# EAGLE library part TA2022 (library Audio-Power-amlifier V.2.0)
STEREO 90W (4.) CLASS-TM DIGITAL AUDIO AMPLIFIER DRIVER USING DIGITAL POWER PROCESSING (DPP TM) TECHNOLOGY Source: http://www.tripath.com/audio.htm .. TA2022.pdf
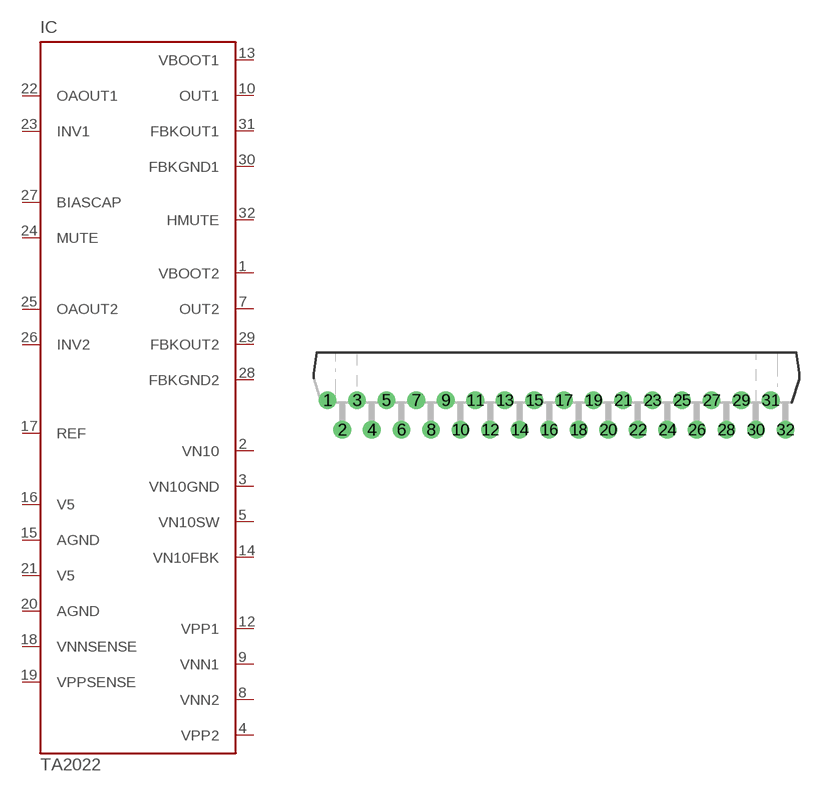
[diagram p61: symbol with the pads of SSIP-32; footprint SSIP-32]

Designator prefix IC

## TA2022 (OC_FARNELL: unknown; OC_NEWARK: unknown)  [SSIP-32]
1  VBOOT2  in
2  VN10  in
3  VN10GND  pwr
4  VPP2  pwr
5  VN10SW  out
7  OUT2  out
8  VNN2  pwr
9  VNN1  pwr
10  OUT1  out
12  VPP1  pwr
13  VBOOT1  in
14  VN10FBK  out
15  AGND  pwr
16  V5  pwr
17  REF  pas
18  VNNSENSE  in
19  VPPSENSE  in
20  AGND  pwr
21  V5  pwr
22  OAOUT1  out
23  INV1  in
24  MUTE  in
25  OAOUT2  out
26  INV2  in
27  BIASCAP  pas
28  FBKGND2  out
29  FBKOUT2  out
30  FBKGND1
31  FBKOUT1  out
32  HMUTE  out

## Footprint SSIP-32 (pad centres in mm)
32-pin SSIP Source: http://www.tripath.com/audio.htm
drill 0.813 pad 1.524: 1 -19.685,2.54; 2 -18.415,0; 3 -17.145,2.54; 4 -15.875,0; 5 -14.605,2.54; 6 -13.335,0; 7 -12.065,2.54; 8 -10.795,0; 9 -9.525,2.54; 10 -8.255,0; 11 -6.985,2.54; 12 -5.715,0; 13 -4.445,2.54; 14 -3.175,0; 15 -1.905,2.54; 16 -0.635,0; 17 0.635,2.54; 18 1.905,0; 19 3.175,2.54; 20 4.445,0; 21 5.715,2.54; 22 6.985,0; 23 8.255,2.54; 24 9.525,0; 25 10.795,2.54; 26 12.065,0; 27 13.335,2.54; 28 14.605,0; 29 15.875,2.54; 30 17.145,0; 31 18.415,2.54; 32 19.685,0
